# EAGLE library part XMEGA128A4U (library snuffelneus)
MICROCONTROLLER Features High-performance, Low-power 8/16-bit AVR XMEGA Microcontroller Non-Volatile Program and Data Memories - 16 KB - 128 KB of In-System Self-Programmable Flash - 4 KB - 8 KB Boot Code Section with Independent Lock Bits - 1 KB - 2 KB EEPROM - 2 KB - 8 KB Internal SRAM Peripheral Features - Four-channel DMA Controller with support for external requests - Eight-channel Event System - Five 16-bit Timer/Counters Three Timer/Counters with 4 Output Compare or Input Capture channels Two Timer/Counters with 2 Output Compare or Input Capture channels High-Resolution Extensions on all Timer/Counters Advanced Waveform Extension on one Timer/Counter - Five USARTs IrDA Extension on one USART - Two Two-Wire Interfaces with dual address match (I2C and SMBus compatible) - Two SPIs (Serial Peripheral Interfaces) peripherals - AES and DES Crypto Engine - 16-bit Real Time Counter with Separate Oscillator - One Twelve-channel, 12-bit, 2 Msps Analog to Digital Converter - One Two-channel, 12-bit, 1 Msps Digital to Analog Converter - Two Analog Comparators with Window compare function - External Interrupts on all General Purpose I/O pins - Programmable Watchdog Timer with Separate On-chip Ultra Low Power Oscillator Special Microcontroller Features - Power-on Reset and Programmable Brown-out Detection - Internal and External Clock Options with PLL - Programmable Multi-level Interrupt Controller - Sleep Modes: Idle, Power-down, Standby, Power-save, Extended Standby - Advanced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
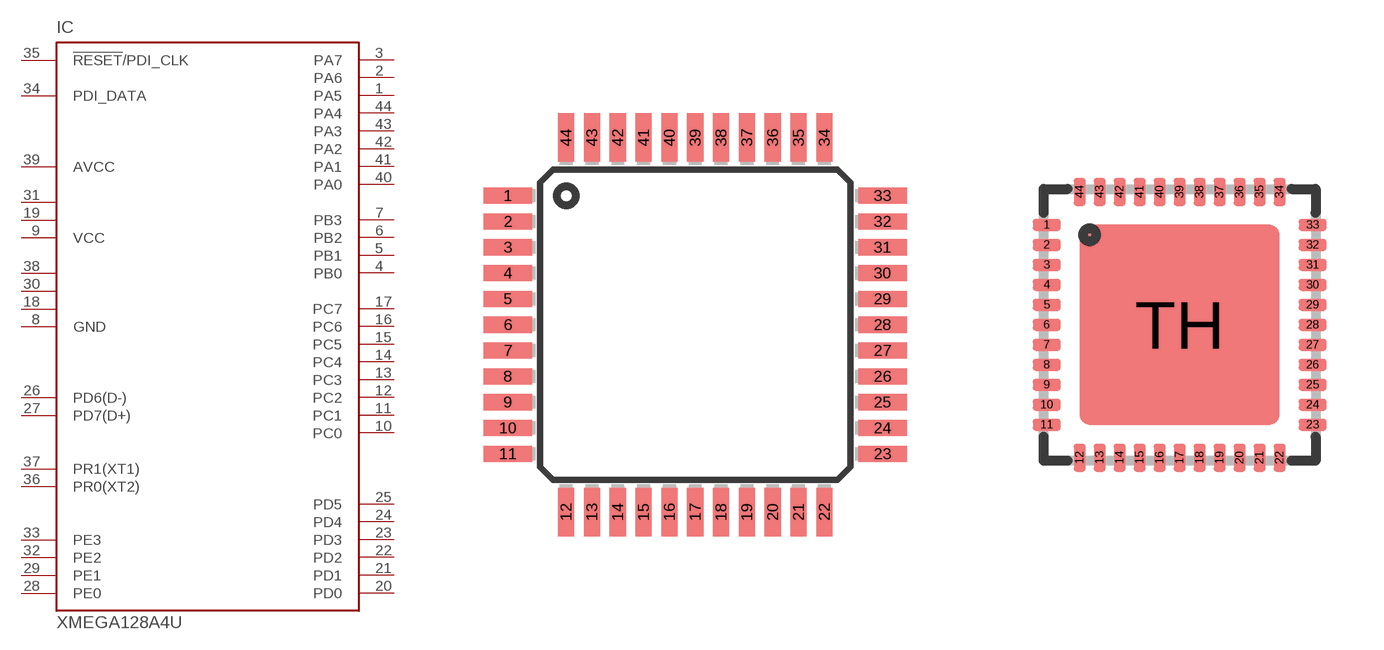
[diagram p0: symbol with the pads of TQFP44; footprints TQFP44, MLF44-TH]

Designator prefix IC

## XMEGA128A4UA (OC_FARNELL: unknown; OC_NEWARK: unknown)  [TQFP44]
1  PA5
2  PA6
3  PA7
4  PB0
5  PB1
6  PB2
7  PB3
8  GND  pwr
9  VCC  pwr
10  PC0
11  PC1
12  PC2
13  PC3
14  PC4
15  PC5
16  PC6
17  PC7
18  GND1  pwr
19  VCC1  pwr
20  PD0
21  PD1
22  PD2
23  PD3
24  PD4
25  PD5
26  PD6(D-)
27  PD7(D+)
28  PE0
29  PE1
30  GND2  pwr
31  VCC2  pwr
32  PE2
33  PE3
34  PDI_DATA
35  !RESET!/PDI_CLK
36  PR0(XT2)
37  PR1(XT1)
38  GND3  pwr
39  AVCC  pwr
40  PA0
41  PA1
42  PA2
43  PA3
44  PA4

## XMEGA128A4UM1 (OC_FARNELL: unknown; OC_NEWARK: unknown)  [MLF44-TH]
Pads as for TQFP44

## Footprint TQFP44 (pad centres in mm)
44-lead Thin Quad Flat Package
smd 1.5 x 0.5: 1 -5.8,4; 2 -5.8,3.2; 3 -5.8,2.4; 4 -5.8,1.6; 5 -5.8,0.8; 6 -5.8,0; 7 -5.8,-0.8; 8 -5.8,-1.6; 9 -5.8,-2.4; 10 -5.8,-3.2; 11 -5.8,-4; 23 5.8,-4; 24 5.8,-3.2; 25 5.8,-2.4; 26 5.8,-1.6; 27 5.8,-0.8; 28 5.8,0; 29 5.8,0.8; 30 5.8,1.6; 31 5.8,2.4; 32 5.8,3.2; 33 5.8,4
smd 0.5 x 1.5: 12 -4,-5.8; 13 -3.2,-5.8; 14 -2.4,-5.8; 15 -1.6,-5.8; 16 -0.8,-5.8; 17 0,-5.8; 18 0.8,-5.8; 19 1.6,-5.8; 20 2.4,-5.8; 21 3.2,-5.8; 22 4,-5.8; 34 4,5.8; 35 3.2,5.8; 36 2.4,5.8; 37 1.6,5.8; 38 0.8,5.8; 39 0,5.8; 40 -0.8,5.8; 41 -1.6,5.8; 42 -2.4,5.8; 43 -3.2,5.8; 44 -4,5.8

## Footprint MLF44-TH (pad centres in mm)
44M1 Micro Lead Frame package (MLF) Source: http://www.atmel.com/dyn/resources/prod_documents/doc2593.pdf
smd 0.7 x 0.3: 1 -3.325,2.5; 2 -3.325,2; 3 -3.325,1.5; 4 -3.325,1; 5 -3.325,0.5; 6 -3.325,0; 7 -3.325,-0.5; 8 -3.325,-1; 9 -3.325,-1.5; 10 -3.325,-2; 11 -3.325,-2.5; 23 3.325,-2.5; 24 3.325,-2; 25 3.325,-1.5; 26 3.325,-1; 27 3.325,-0.5; 28 3.325,0; 29 3.325,0.5; 30 3.325,1; 31 3.325,1.5; 32 3.325,2; 33 3.325,2.5
smd 0.3 x 0.7: 12 -2.5,-3.325; 13 -2,-3.325; 14 -1.5,-3.325; 15 -1,-3.325; 16 -0.5,-3.325; 17 0,-3.325; 18 0.5,-3.325; 19 1,-3.325; 20 1.5,-3.325; 21 2,-3.325; 22 2.5,-3.325; 34 2.5,3.325; 35 2,3.325; 36 1.5,3.325; 37 1,3.325; 38 0.5,3.325; 39 0,3.325; 40 -0.5,3.325; 41 -1,3.325; 42 -1.5,3.325; 43 -2,3.325; 44 -2.5,3.325
smd 5 x 5: TH 0,0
